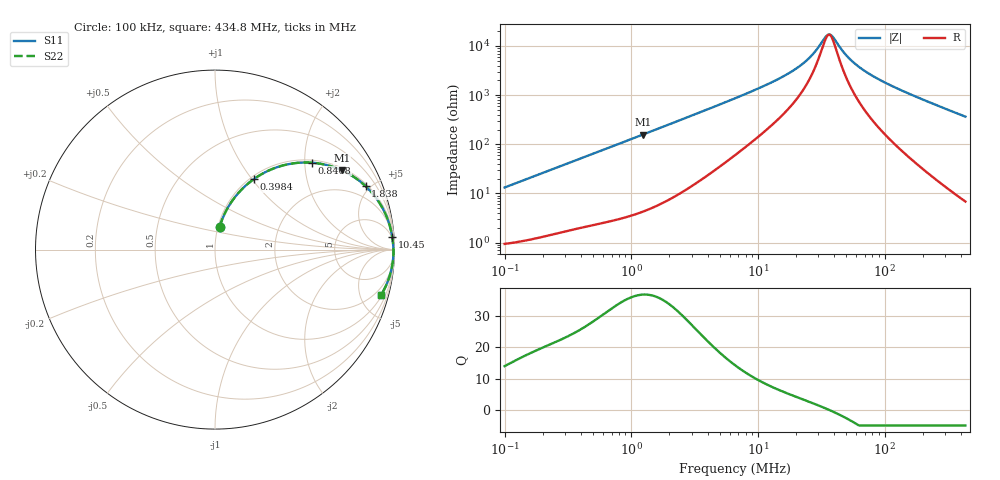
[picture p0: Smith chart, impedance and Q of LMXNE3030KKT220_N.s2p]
! LMXNE3030KKT220_N  S-PARAMETER MODEL  ( General Type )
! Model Generated by TAIYO YUDEN Corporation (http://www.ty-top.com)
! Version 1.0
! TAIYO YUDEN Control No. 191023NI43SB-FBB
! Copyright(c) 2019 TAIYO YUDEN CO.,LTD. All Rights Reserved.
! Product Description (link to TY-COMPAS)
! https://ds.yuden.co.jp/TYCOMPAS/or/detail?pn=LMXNE3030KKT220MN&u=M
! Products Name : Inductors
! Characteristics :
!  Inductance : 22 uH , SRF(min) : 22 MHz , DC Resistance(max) : 0.924 Ohm
!  Rated Current : Saturation :380 mA , Temp Rise : 410 mA
!  Case Size : 3.0 x 3.0 / 0.118 x 0.118 [mm/inch] , Thickness : 1 / 0.039 [mm/inch]
!  (Conditions: Temperature = 25 degC , DC Bias Current/Voltage = 0A / 0V)
! External Node Assignments :
!  1  o---GGG---o  2
! GND o---------o GND
! Frequency Range : 0.1MHz  -  434.768421MHz  [ 402 STEP ]
# MHz S RI R 50
! Freq[MHz].  S11 Real  S11 Imag  S21 Real  S21 Imag  S12 Real  S12 Imag  S22 Real  S22 Imag
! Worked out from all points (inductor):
!   401 points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, 100 kHz to 434.8 MHz, reference 50 ohm
!   read as one part in series: L = 21 uH near 104.3 kHz
!   highest Q = 36.9 at 1.234 MHz (marker M1), where L = 20.3 uH
!   self-resonance near 35.96 MHz
!   S11 on the Smith chart (normalised r, x): 100 kHz: 1.02, +0.26; 398.4 kHz: 1.04, +1.03; 846.8 kHz: 1.06, +2.17; 1.838 MHz: 1.13, +4.69; 10.45 MHz: 4, +28; 434.8 MHz: 1.14, -7.30
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0.1  0.026 0.1274  0.974 -0.1274  0.974 -0.1274  0.026 0.1274
0.21704  0.0853 0.2561  0.9147 -0.2561  0.9147 -0.2561  0.0853 0.2561
0.398394  0.2186 0.3943  0.7814 -0.3943  0.7814 -0.3943  0.2186 0.3943
0.406826  0.2253 0.399  0.7747 -0.399  0.7747 -0.399  0.2253 0.399
0.605655  0.3806 0.4695  0.6194 -0.4695  0.6194 -0.4695  0.3806 0.4695
0.846751  0.5389 0.4843  0.4611 -0.4843  0.4611 -0.4843  0.5389 0.4843
1.234461  0.708 0.4414  0.292 -0.4414  0.292 -0.4414  0.708 0.4414
1.65507  0.8103 0.3784  0.1897 -0.3784  0.1897 -0.3784  0.8103 0.3784
1.837785  0.8393 0.3532  0.1607 -0.3532  0.1607 -0.3532  0.8393 0.3532
3.167973  0.935 0.2281  0.065 -0.2281  0.065 -0.2281  0.935 0.2281
6.733248  0.9796 0.11  0.0204 -0.11  0.0204 -0.11  0.9796 0.11
10.45281  0.9877 0.0683  0.0123 -0.0683  0.0123 -0.0683  0.9877 0.0683
18.78933  0.9923 0.031  0.00773 -0.031  0.00773 -0.031  0.9923 0.031
26.82484  0.9936 0.0137  0.00642 -0.0137  0.00642 -0.0137  0.9936 0.0137
34.48935  0.9941 0.00241  0.00588 -0.00241  0.00588 -0.00241  0.9941 0.00241
37.50313  0.9942 -0.00132  0.00576 0.00132  0.00576 0.00132  0.9942 -0.00132
49.23919  0.9944 -0.0138  0.00561 0.0138  0.00561 0.0138  0.9944 -0.0138
58.22052  0.9943 -0.0219  0.00573 0.0219  0.00573 0.0219  0.9943 -0.0219
76.43979  0.9936 -0.0367  0.00637 0.0367  0.00637 0.0367  0.9936 -0.0367
109.1303  0.9915 -0.0604  0.0085 0.0604  0.0085 0.0604  0.9915 -0.0604
222.432  0.9771 -0.1334  0.0229 0.1334  0.0229 0.1334  0.9771 -0.1334
434.7684  0.9261 -0.2523  0.0739 0.2523  0.0739 0.2523  0.9261 -0.2523
